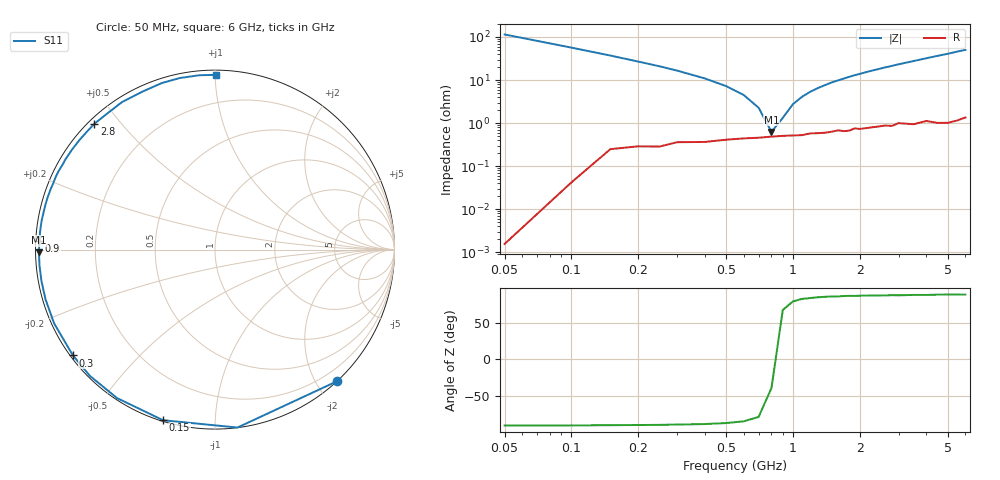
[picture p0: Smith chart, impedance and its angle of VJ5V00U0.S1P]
! Infineon Technologies  Discrete & RF Semiconductors
! BB 914
! Si Tuning Diode in SOT23
! VR = 5 V
! S-Parameters:  July  1999
# GHz  S  MA  R  50
!  f  S11
! GHz  MAG  ANG
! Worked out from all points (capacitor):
!   34 points, 50 MHz to 6 GHz, reference 50 ohm
!   read as one part to ground: C = 27.7 pF near 50 MHz
!   lowest |Z| = 624 mohm at 800 MHz (marker M1)
!   series resonance near 824.3 MHz, so ESL is about 1.3 nH
!   S11 on the Smith chart (normalised r, x): 50 MHz: 0.00, -2.29; 150 MHz: 0.00, -0.74; 300 MHz: 0.01, -0.33; 900 MHz: 0.01, +0.02; 2.8 GHz: 0.02, +0.43; 6 GHz: 0.03, +1.00
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0.05  1 -47.2
0.1  0.9993 -82.8
0.15  0.9936 -106.9
0.2  0.9911 -123.4
0.25  0.9903 -134.7
0.3  0.9871 -143.3
0.4  0.9862 -155.4
0.5  0.984 -163.6
0.6  0.9827 -169.8
0.7  0.9819 -174.9
0.8  0.9808 -179.1
0.9  0.98 177.2
1  0.9796 173.8
1.2  0.9774 167.8
1.5  0.9758 160.0
1.6  0.9742 157.8
1.9  0.9721 151.0
2.2  0.972 144.8
2.4  0.971 141.1
2.6  0.9701 137.2
2.8  0.9712 133.8
3  0.9677 130.2
3.5  0.9716 122.2
4  0.9688 114.6
4.5  0.974 107.7
5  0.9759 101.6
5.5  0.9754 95.1
6  0.9734 89.8
